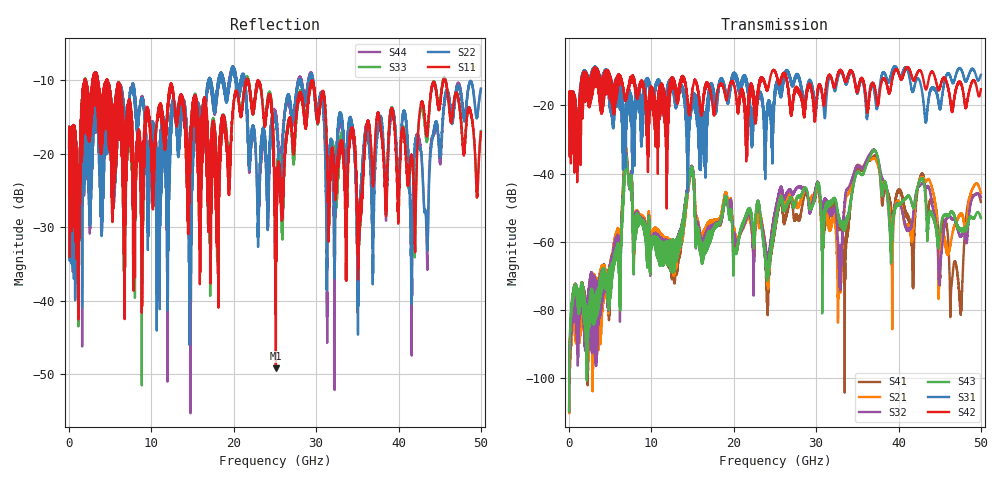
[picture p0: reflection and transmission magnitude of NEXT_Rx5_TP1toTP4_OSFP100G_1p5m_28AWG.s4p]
! Touchstone data
! Created: 27-Feb-2019 by IdEM 12 (12.1.0)
! COMMENTS
!  Created Wed Feb 27 09:43:39 2019
!  64 Port Network Data from SP1.SP block
!  freq  magS1_1  angS1_1  magS1_2  angS1_2  magS1_3  angS1_3  magS1_4  angS1_4
!  magS1_5  angS1_5  magS1_6  angS1_6  magS1_7  angS1_7  magS1_8  angS1_8
!  magS1_9  angS1_9  magS1_10  angS1_10  magS1_11  angS1_11  magS1_12  angS1_12
!  magS1_13  angS1_13  magS1_14  angS1_14  magS1_15  angS1_15  magS1_16  angS1_16
!  magS1_17  angS1_17  magS1_18  angS1_18  magS1_19  angS1_19  magS1_20  angS1_20
!  magS1_21  angS1_21  magS1_22  angS1_22  magS1_23  angS1_23  magS1_24  angS1_24
!  magS1_25  angS1_25  magS1_26  angS1_26  magS1_27  angS1_27  magS1_28  angS1_28
!  magS1_29  angS1_29  magS1_30  angS1_30  magS1_31  angS1_31  magS1_32  angS1_32
!  magS1_33  angS1_33  magS1_34  angS1_34  magS1_35  angS1_35  magS1_36  angS1_36
!  magS1_37  angS1_37  magS1_38  angS1_38  magS1_39  angS1_39  magS1_40  angS1_40
!  magS1_41  angS1_41  magS1_42  angS1_42  magS1_43  angS1_43  magS1_44  angS1_44
!  magS1_45  angS1_45  magS1_46  angS1_46  magS1_47  angS1_47  magS1_48  angS1_48
!  magS1_49  angS1_49  magS1_50  angS1_50  magS1_51  angS1_51  magS1_52  angS1_52
!  magS1_53  angS1_53  magS1_54  angS1_54  magS1_55  angS1_55  magS1_56  angS1_56
!  magS1_57  angS1_57  magS1_58  angS1_58  magS1_59  angS1_59  magS1_60  angS1_60
!  magS1_61  angS1_61  magS1_62  angS1_62  magS1_63  angS1_63  magS1_64  angS1_64
!  magS2_1  angS2_1  magS2_2  angS2_2  magS2_3  angS2_3  magS2_4  angS2_4
!  magS2_5  angS2_5  magS2_6  angS2_6  magS2_7  angS2_7  magS2_8  angS2_8
!  magS2_9  angS2_9  magS2_10  angS2_10  magS2_11  angS2_11  magS2_12  angS2_12
!  magS2_13  angS2_13  magS2_14  angS2_14  magS2_15  angS2_15  magS2_16  angS2_16
!  magS2_17  angS2_17  magS2_18  angS2_18  magS2_19  angS2_19  magS2_20  angS2_20
!  magS2_21  angS2_21  magS2_22  angS2_22  magS2_23  angS2_23  magS2_24  angS2_24
!  magS2_25  angS2_25  magS2_26  angS2_26  magS2_27  angS2_27  magS2_28  angS2_28
!  magS2_29  angS2_29  magS2_30  angS2_30  magS2_31  angS2_31  magS2_32  angS2_32
!  magS2_33  angS2_33  magS2_34  angS2_34  magS2_35  angS2_35  magS2_36  angS2_36
!  magS2_37  angS2_37  magS2_38  angS2_38  magS2_39  angS2_39  magS2_40  angS2_40
!  magS2_41  angS2_41  magS2_42  angS2_42  magS2_43  angS2_43  magS2_44  angS2_44
!  magS2_45  angS2_45  magS2_46  angS2_46  magS2_47  angS2_47  magS2_48  angS2_48
!  magS2_49  angS2_49  magS2_50  angS2_50  magS2_51  angS2_51  magS2_52  angS2_52
!  magS2_53  angS2_53  magS2_54  angS2_54  magS2_55  angS2_55  magS2_56  angS2_56
!  magS2_57  angS2_57  magS2_58  angS2_58  magS2_59  angS2_59  magS2_60  angS2_60
!  magS2_61  angS2_61  magS2_62  angS2_62  magS2_63  angS2_63  magS2_64  angS2_64
!  magS3_1  angS3_1  magS3_2  angS3_2  magS3_3  angS3_3  magS3_4  angS3_4
!  magS3_5  angS3_5  magS3_6  angS3_6  magS3_7  angS3_7  magS3_8  angS3_8
!  magS3_9  angS3_9  magS3_10  angS3_10  magS3_11  angS3_11  magS3_12  angS3_12
!  magS3_13  angS3_13  magS3_14  angS3_14  magS3_15  angS3_15  magS3_16  angS3_16
!  magS3_17  angS3_17  magS3_18  angS3_18  magS3_19  angS3_19  magS3_20  angS3_20
!  magS3_21  angS3_21  magS3_22  angS3_22  magS3_23  angS3_23  magS3_24  angS3_24
!  magS3_25  angS3_25  magS3_26  angS3_26  magS3_27  angS3_27  magS3_28  angS3_28
!  magS3_29  angS3_29  magS3_30  angS3_30  magS3_31  angS3_31  magS3_32  angS3_32
!  magS3_33  angS3_33  magS3_34  angS3_34  magS3_35  angS3_35  magS3_36  angS3_36
!  magS3_37  angS3_37  magS3_38  angS3_38  magS3_39  angS3_39  magS3_40  angS3_40
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# Hz S MA R 50
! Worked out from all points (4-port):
!   5000 points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, 10 MHz to 50 GHz, reference 50 ohm
!   strongest paths, dB at 10 MHz, 12.51 GHz, 25.01 GHz, 37.51 GHz, 50 GHz:
!     S42: -19.6, -13.2, -10.0, -20.0, -15.2
!     S31: -19.6, -14.0, -15.9, -19.1, -11.0
!     S43: -109.8, -65.7, -55.1, -35.8, -53.1
!     S32: -109.8, -65.9, -51.9, -35.8, -47.0
!     S21: -108.0, -65.2, -52.1, -37.7, -45.8
!     S41: -109.2, -64.9, -55.6, -37.0, -48.3
!   lowest |S11| = -49.2 dB at 25.11 GHz (marker M1), VSWR 1.01, Z = 50.3 + j0.113 ohm
!   |S11| at or under -10 dB: 4.66 GHz to 21.51 GHz (16.85 GHz wide, 129 % of centre); 22.94 GHz to 45.47 GHz (22.53 GHz wide, 65.9 % of centre); 45.68 GHz to end of sweep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
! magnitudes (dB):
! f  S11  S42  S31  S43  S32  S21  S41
! 10 MHz  -19.2  -19.6  -19.6  -109.8  -109.8  -108.0  -109.2
! 6.94 GHz  -17.5  -17.7  -19.7  -34.7  -33.8  -32.4  -33.2
! 25.11 GHz  -49.2  -10.6  -14.8  -53.6  -50.4  -50.7  -54.2
! 32.8 GHz  -18.9  -10.1  -10.8  -53.2  -65.0  -71.9  -55.2
! 42.87 GHz  -12.9  -10.8  -16.2  -41.4  -42.8  -41.0  -40.1
! 47.51 GHz  -14.6  -13.4  -9.3  -56.9  -58.4  -52.1  -80.7
! 50 GHz  -17.1  -15.2  -11.0  -53.1  -47.0  -45.8  -48.3
